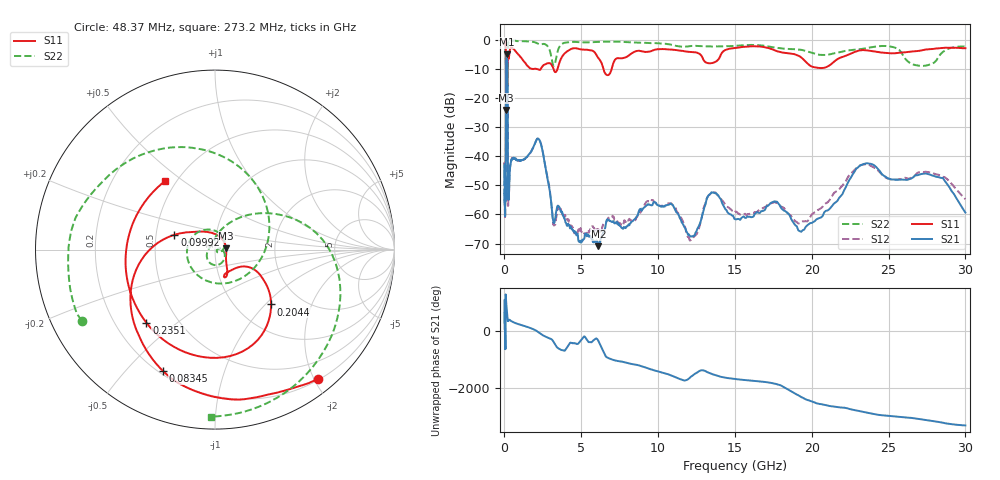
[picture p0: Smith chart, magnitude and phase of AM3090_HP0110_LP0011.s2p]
! Date/Time: Thu, Feb 28, 2019 1:59 PM
! Network Analyzer: Agilent Technologies E8364B Rev: A.07.50.67
! Sweep from 0.010 to 30.000 GHz, 1601 Points, Sweep Type: LOG
! Power Supply: 5.023 V, 0.002 A
# Hz S DB R 50
!freq MagS11 AngS11 MagS21 AngS21 MagS12 AngS12 MagS22 AngS22
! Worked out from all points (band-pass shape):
!   1601 points, 10 MHz to 30 GHz, reference 50 ohm
!   highest |S21| = -4.90 dB at 146.9 MHz (marker M1); lowest = -70.9 dB at 6.11 GHz (marker M2)
!   |S21| within 3 dB of the highest: 109.6 MHz to 189.1 MHz (79.51 MHz wide, 53.2 % of centre)
!   lowest |S11| = -24.1 dB at 107.7 MHz (marker M3), VSWR 1.13, Z = 56.6 + j0.927 ohm
!   |S11| at or under -10 dB: 2.148 GHz to 2.359 GHz (211.6 MHz wide, 9.39 % of centre); 3.197 GHz to 3.453 GHz (255.7 MHz wide, 7.69 % of centre); 6.447 GHz to 6.977 GHz (529.4 MHz wide, 7.89 % of centre)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
!   |S22| runs from -39.9 to -0.2 dB; largest |S21 - S12| = 0.013
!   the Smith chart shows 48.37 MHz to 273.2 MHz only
!   S11 on the Smith chart (normalised r, x): 48.37 MHz: 0.22, -2.05; 83.45 MHz: 0.22, -0.64; 99.92 MHz: 0.62, +0.11; 204.4 MHz: 1.43, -1.08; 235.1 MHz: 0.33, -0.39; 273.2 MHz: 0.44, +0.43
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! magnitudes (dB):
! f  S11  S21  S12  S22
! 10 MHz  -0.3  -49.8  -43.0  -0.6
! 38.04 MHz  -0.5  -60.0  -59.1  -1.4
! 48.37 MHz  -0.7  -48.0  -49.9  -1.5
! 83.45 MHz  -2.7  -48.4  -49.0  -5.6
! 99.92 MHz  -12.4  -16.0  -16.0  -15.1
! 107.7 MHz  -24.1  -8.7  -8.7  -17.3
! 134.2 MHz  -16.1  -5.1  -5.1  -39.9
! 144.7 MHz  -16.8  -4.9  -4.9  -27.4
! 146.9 MHz  -16.8  -4.9  -4.9  -25.3
! 180.3 MHz  -14.8  -6.4  -6.4  -30.0
! 204.4 MHz  -7.2  -18.0  -18.0  -9.3
! 235.1 MHz  -5.1  -53.8  -57.0  -1.4
! 273.2 MHz  -6.5  -54.4  -53.9  -0.6
! 550.5 MHz  -2.9  -40.7  -40.7  -0.2
! 2.084 GHz  -9.9  -34.4  -34.4  -1.0
! 3.22 GHz  -10.4  -63.0  -63.8  -8.9
! 6.11 GHz  -6.2  -70.9  -65.3  -0.6
! 7.926 GHz  -5.9  -64.2  -62.3  -0.7
! 13.61 GHz  -7.8  -52.5  -52.3  -2.2
! 19.61 GHz  -7.5  -64.3  -62.3  -3.8
! 23.59 GHz  -3.6  -42.4  -42.7  -2.8
! 30 GHz  -2.8  -59.3  -54.7  -2.2
